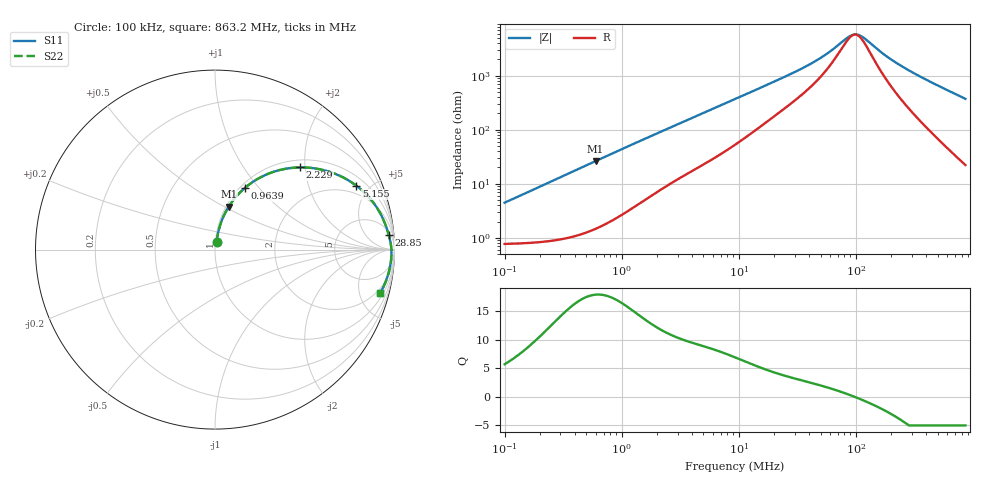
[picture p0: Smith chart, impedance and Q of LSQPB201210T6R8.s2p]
! LSQPB201210T6R8  S-PARAMETER MODEL  ( General Type )
! Model Generated by TAIYO YUDEN Corporation (http://www.ty-top.com)
! Version 2.0
! TAIYO YUDEN Control No. 100810NF18SB-HKC
! Copyright(c) 2007 TAIYO YUDEN CO.,LTD. All Rights Reserved.
! Product Description (link to TY-COMPAS)
! https://ds.yuden.co.jp/TYCOMPAS/or/detail?pn=LSQPB201210T6R8M&u=M
! Products Name : Inductors
! Characteristics :
!  Inductance : 6.8 uH , SRF(min) : 60 MHz , DC Resistance(max) : 0.975 Ohm
!  Rated Current : Saturation :290 mA , Temp Rise : 350 mA (40 degC)
!  Case Size : 2.0 x 1.25 / 0.079 x 0.049 [mm/inch] , Thickness : 1.0 / 0.04 [mm/inch]
!  (Conditions: Temperature = 25 degC , DC Bias Current/Voltage = 0A / 0V)
! External Node Assignments :
!  1  o---GGG---o  2
! GND o---------o GND
! Frequency Range : 0.1MHz  -  863.231078MHz  [ 402 STEP ]
# MHz S RI R 50
! Freq[MHz].  S11 Real  S11 Imag  S21 Real  S21 Imag  S12 Real  S12 Imag  S22 Real  S22 Imag
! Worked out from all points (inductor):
!   401 points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, 100 kHz to 863.2 MHz, reference 50 ohm
!   read as one part in series: L = 7 uH near 104.6 kHz
!   highest Q = 17.9 at 598.9 kHz (marker M1), where L = 6.97 uH
!   self-resonance near 97.97 MHz
!   S11 on the Smith chart (normalised r, x): 100 kHz: 1.02, +0.09; 963.9 kHz: 1.05, +0.84; 2.229 MHz: 1.16, +1.88; 5.155 MHz: 1.47, +4.15; 28.85 MHz: 7, +21; 863.2 MHz: 1.44, -7.45
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0.1  0.00953 0.0432  0.9905 -0.0432  0.9905 -0.0432  0.00953 0.0432
0.226074  0.018 0.0968  0.982 -0.0968  0.982 -0.0968  0.018 0.0968
0.456353  0.0488 0.1882  0.9512 -0.1882  0.9512 -0.1882  0.0488 0.1882
0.598942  0.0762 0.2388  0.9238 -0.2388  0.9238 -0.2388  0.0762 0.2388
0.9639  0.1645 0.3419  0.8355 -0.3419  0.8355 -0.3419  0.1645 0.3419
1.482511  0.303 0.4251  0.697 -0.4251  0.697 -0.4251  0.303 0.4251
2.082584  0.4444 0.4568  0.5556 -0.4568  0.5556 -0.4568  0.4444 0.4568
2.229069  0.4741 0.4581  0.5259 -0.4581  0.5259 -0.4581  0.4741 0.4581
3.276491  0.6365 0.4339  0.3635 -0.4339  0.3635 -0.4339  0.6365 0.4339
5.154841  0.7883 0.3556  0.2117 -0.3556  0.2117 -0.3556  0.7883 0.3556
9.291023  0.902 0.2337  0.098 -0.2337  0.098 -0.2337  0.902 0.2337
16.0041  0.9472 0.1447  0.0528 -0.1447  0.0528 -0.1447  0.9472 0.1447
28.84559  0.968 0.081  0.032 -0.081  0.032 -0.081  0.968 0.081
42.3999  0.9754 0.0513  0.0246 -0.0513  0.0246 -0.0513  0.9754 0.0513
58.22765  0.9795 0.0307  0.0205 -0.0307  0.0205 -0.0307  0.9795 0.0307
85.58835  0.9824 0.00785  0.0176 -0.00785  0.0176 -0.00785  0.9824 0.00785
98.05203  0.983 -4.87e-05  0.017 4.87e-05  0.017 4.87e-05  0.983 -4.87e-05
104.9488  0.9832 -0.00403  0.0168 0.00403  0.0168 0.00403  0.9832 -0.00403
114.905  0.9834 -0.00939  0.0166 0.00939  0.0166 0.00939  0.9834 -0.00939
193.4934  0.9824 -0.0435  0.0176 0.0435  0.0176 0.0435  0.9824 -0.0435
364.9178  0.974 -0.1018  0.026 0.1018  0.026 0.1018  0.974 -0.1018
863.2311  0.9205 -0.2424  0.0795 0.2424  0.0795 0.2424  0.9205 -0.2424
